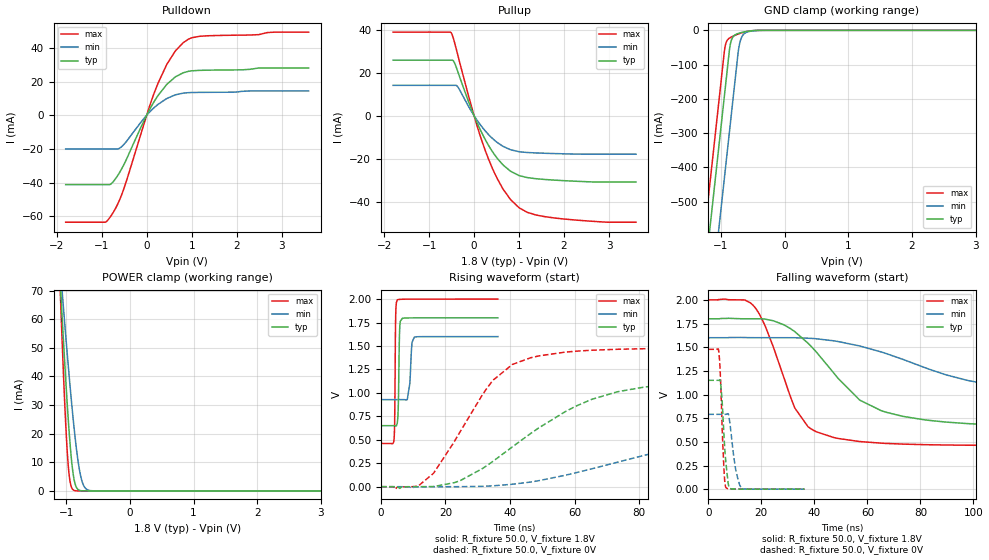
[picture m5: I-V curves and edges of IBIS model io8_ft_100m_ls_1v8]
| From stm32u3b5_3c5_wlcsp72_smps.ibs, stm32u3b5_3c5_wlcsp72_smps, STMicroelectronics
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[Model]   io8_ft_100m_ls_1v8
Model_type I/O
Polarity   Non-Inverting
Enable   Active-Low
| CAP_THRESHOLD on pad IOFT is "UDTCAPC" :
| Rising=30.0% of vddiom   Falling=70.0% of vddiom
| C_comp min and max val. don't necessarily correlate with the min and max pvt
| but are the smallest and greatest pad capacitance found.
| var   typ   min   max
C_comp   3.41155pF  3.41004pF  3.47580pF
|C_comp_pullup   1.91831pF  1.83531pF  2.09497pF
|C_comp_pulldown   1.49324pF  1.57473pF  1.38082pF
Vinl = 800.0mV
Vinh = 1.0V
Vmeas = 900.0mV   | Reference voltage for timing measurements
Cref  = 50.0pF   | Timing specification test load capacitance value
Rref  = 1.0MOhm   | Timing specification test load resistance value
Vref  = 990.0mV   | Timing specification test load voltage
[Model Spec]
| TIME_THRESHOLD on pin ZIV11 is "CMOS" :
| Rising=50.0% of vdd   Falling=50.0% of vdd
Vinl 694.50000mV 619.50000mV 778.50000mV
Vinh 1.08350V 957.50000mV 1.18750V
| variable   typ   min   max
[Temperature Range] 25.0 130.0 -40.0
| variable   typ   min   max
[Voltage Range] 1.8V 1.6V 2.0V
| variable   typ   min   max
[POWER Clamp Reference] 1.8V 1.6V 2.0V
| variable   typ   min   max
[GND Clamp Reference] 0V 0V 0V
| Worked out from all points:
|   slope of the pulldown table from 0 to 0.27 V, typ, clamps not added: 21.9 ohm
|   slope of the pullup table from 0 to 0.27 V, typ, clamps not added: 22.7 ohm
|   GND clamp passes 1 mA (typ) near -0.50 V on its own axis
|   POWER clamp passes 1 mA (typ) near -0.83 V on its own axis
|   rising waveform, R_fixture 50.0, V_fixture 1.8V: 20-80 % time 317ps typ, 692ps min, 233ps max; typ from 0.65 V to 1.8 V
|   falling waveform, R_fixture 50.0, V_fixture 1.8V: 20-80 % time 25ns typ, 53.7ns min, 13ns max; typ from 1.8 V to 0.65 V
|   rising waveform, R_fixture 50.0, V_fixture 0V: 20-80 % time 31.5ns typ, 66.4ns min, 17.2ns max; typ from 0 V to 1.15 V
|   falling waveform, R_fixture 50.0, V_fixture 0V: 20-80 % time 1.6ns typ, 2.32ns min, 1.18ns max; typ from 1.15 V to 0 V
[POWER Clamp]
-1.8V     399.1mA    292.1mA    557.7mA
-1.09V    71.2mA     76.8mA     67.14mA
-1.08V    67.05mA    73.98mA    61.2mA
-1.06V    58.89mA    68.38mA    49.67mA
-1.02V    43.22mA    57.4mA     28.67mA
-980mV    28.81mA    46.77mA    12.28mA
-940mV    16.45mA    36.61mA    3.257mA
-880mV    4.35mA     22.67mA    225.4uA
-820mV    610.4uA    11.29mA    13uA
-770mV    97.5uA     4.87mA     1.193uA
-640mV    753.9nA    196uA      2.499nA
3.6V      0A         0A         0A
[GND Clamp]
-1.8V     -1.64A     -1.88A     -1.509A
-1.24V    -688.2mA   -927.9mA   -557mA
-1.05V    -365.2mA   -604.9mA   -234mA
-950mV    -195.2mA   -434.9mA   -64mA
-930mV    -161.2mA   -400.9mA   -41.59mA
-870mV    -59.19mA   -298.9mA   -22.94mA
-850mV    -36.73mA   -264.9mA   -20.65mA
-770mV    -12.21mA   -128.9mA   -13.73mA
-730mV    -9.139mA   -62.1mA    -10.81mA
-690mV    -6.97mA    -26.33mA   -8.198mA
-530mV    -1.564mA   -2.413mA   -1.407mA
3.6V      1.23nA     159nA      530.1pA
| variable   typ   min   max
[Pullup Reference] 1.8V 1.6V 2.0V
| variable   typ   min   max
[Pulldown Reference] 0V 0V 0V
[Pullup]
-1.8V     25.8mA     14.11mA    38.84mA
-510mV    25.8mA     14.11mA    38.55mA
-450mV    25.15mA    14.11mA    35.19mA
-370mV    20.99mA    13.61mA    28.84mA
20mV      -1.001mA   -644.5uA   -1.446mA
300mV     -13.02mA   -8.285mA   -19mA
450mV     -17.96mA   -11.34mA   -26.42mA
650mV     -23mA      -14.3mA    -34.27mA
1V        -27.82mA   -16.74mA   -42.77mA
1.37V     -29.26mA   -17.3mA    -46.1mA
1.74V     -29.87mA   -17.57mA   -47.39mA
3.6V      -30.8mA    -17.88mA   -49.48mA
[Pulldown]
-1.8V     -41.16mA   -19.96mA   -63.43mA
-920mV    -41.16mA   -19.96mA   -63.43mA
-780mV    -40.43mA   -19.96mA   -59.18mA
-620mV    -34.74mA   -19.77mA   -51.3mA
-510mV    -29.46mA   -17.38mA   -43.8mA
0V        0A         0A         0A
250mV     11.64mA    6.428mA    18.87mA
460mV     18.67mA    10.12mA    30.76mA
630mV     22.61mA    12.05mA    37.86mA
810mV     25.21mA    13.14mA    43.03mA
1.18V     26.67mA    13.59mA    46.9mA
3.6V      28.11mA    14.46mA    49.37mA
[Ramp]
dV/dt_r 690.00871mV/31.4598ns 474.20407mV/66.22981ns 886.36378mV/16.51496ns
dV/dt_f 689.75456mV/24.21664ns 402.84322mV/53.30618ns 923.68065mV/12.2716ns
R_load = 50.0
| Removed startup time: 0s 0s 0s  .
| Removed end time: 36.25ns.
[Rising Waveform]
R_fixture   = 50.0
V_fixture   = 1.8V
V_fixture_min = 1.6V
V_fixture_max = 2.0V
0s        650.4mV    928.3mV    460.5mV
4ns       650.4mV    928.3mV    486.7mV
4.25ns    650.2mV    928.3mV    692.9mV
4.6ns     647.8mV    928.3mV    1.858V
5.05ns    677.5mV    928.3mV    1.989V
5.85ns    1.712V     928.3mV    1.997V
6.65ns    1.795V     928.4mV    1.998V
8.15ns    1.799V     927.3mV    1.999V
10.35ns   1.799V     1.594V     1.999V
36.25ns   1.8V       1.6V       2V
| Removed startup time: 0s 0s 0s  .
| Removed end time: 399.25ns.
[Falling Waveform]
R_fixture   = 50.0
V_fixture   = 1.8V
V_fixture_min = 1.6V
V_fixture_max = 2.0V
0s        1.8V       1.6V       2V
16.75ns   1.8V       1.6V       1.946V
21.65ns   1.795V     1.6V       1.709V
32.6ns    1.664V     1.6V       857.9mV
37.6ns    1.542V     1.595V     659.2mV
57.05ns   942.2mV    1.513V     503.4mV
81.5ns    732.8mV    1.285V     470.2mV
106ns     681.1mV    1.105V     462.9mV
138.6ns   659.7mV    1.008V     460.9mV
399.3ns   650.4mV    928.6mV    460.5mV
| Removed startup time: 0s 0s 0s  .
| Removed end time: 399.2ns.
[Rising Waveform]
R_fixture   = 50.0
V_fixture   = 0V
V_fixture_min = 0V
V_fixture_max = 0V
0s        4.649nV    97.48nV    3.434nV
11.65ns   -319.1uV   -264.2uV   9.995mV
16.3ns    1.46mV     -144.3uV   143mV
34.85ns   273.8mV    9.605mV    1.139V
40.75ns   425.4mV    26.25mV    1.303V
57.05ns   798.8mV    121.5mV    1.434V
73.35ns   1.012V     261.8mV    1.465V
88.3ns    1.087V     390.3mV    1.473V
154.8ns   1.147V     714mV      1.477V
399.2ns   1.15V      790.3mV    1.477V
| Removed startup time: 0s 0s 0s  .
| Removed end time: 36.25ns.
[Falling Waveform]
R_fixture   = 50.0
V_fixture   = 0V
V_fixture_min = 0V
V_fixture_max = 0V
0s        1.15V      790.6mV    1.477V
3.9ns     1.15V      790.6mV    1.459V
4.35ns    1.156V     790.6mV    1.309V
4.85ns    1.053V     790.6mV    972.4mV
5.85ns    593.2mV    790.6mV    231.4mV
6.65ns    272.6mV    790.6mV    15.13mV
8.15ns    7.867mV    694.2mV    1.814mV
10.35ns   1.024mV    202.6mV    812uV
12.6ns    490.2uV    7.945mV    625.6uV
36.25ns   214.3uV    165uV      119.6uV
